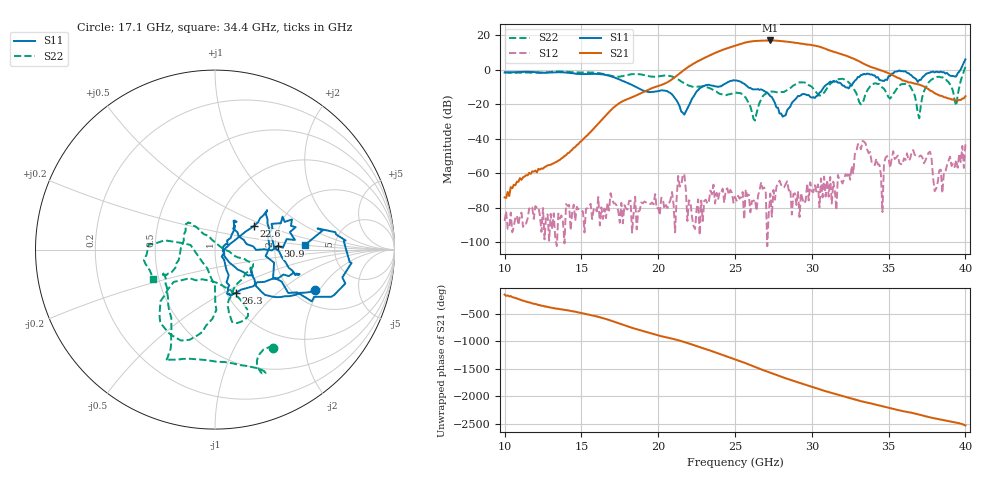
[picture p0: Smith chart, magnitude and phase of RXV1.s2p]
!Keysight Technologies,M9808A,MY58100618,A.14.70.03
!Date: Monday, February 27, 2023 13:25:10
!Correction: S11(Cdelta 2-Port  )
!S21(Cdelta 2-Port  )
!S12(Cdelta 2-Port  )
!S22(Cdelta 2-Port  )
!S2P File: Measurements: S11, S21, S12, S22:
# Hz S  RI  R 50
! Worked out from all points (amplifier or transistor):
!   301 points, 10 GHz to 40 GHz, reference 50 ohm
!   highest |S21| = 16.9 dB at 27.3 GHz (marker M1)
!   |S21| within 3 dB of that: 25.01 GHz to 30.24 GHz (5.222 GHz wide, 18.9 % of centre)
!   unconditionally stable (mu >= 1): start of sweep to 39.64 GHz
!   at 15 GHz: K = 99719.20, MAG = -32.9 dB, |S12| = -81.6 dB
!   at 25 GHz: K = 358.96, MAG = 15.2 dB, |S12| = -73.7 dB
!   at 40 GHz: K = 566.44, MSG = 14.0 dB, |S12| = -43.4 dB
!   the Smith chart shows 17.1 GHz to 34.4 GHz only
!   S11 on the Smith chart (normalised r, x): 17.1 GHz: 2.58, -1.83; 22.6 GHz: 1.48, +0.42; 26.3 GHz: 1.10, -0.57; 30.9 GHz: 2.07, +0.10; 34.4 GHz: 3.02, +0.23
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1e10  0.1017 0.8226  -0.000174 -9.79e-05  1.08e-07 -4.14e-05  0.6897 0.4632
1.5e10  0.7404 0.0739  -0.00493 -0.00703  7.26e-05 4.13e-05  0.6592 -0.495
1.71e10  0.5569 -0.2259  0.0154 0.0785  0.000134 1.4e-05  0.3258 -0.5456
2e10  0.2012 -0.1266  -0.3335 -0.0387  -8.62e-05 -5.11e-05  -0.1776 -0.6089
2.26e10  0.2175 0.1331  1.697 -0.4654  0.000171 3.16e-05  -0.293 -0.1269
2.38e10  0.3004 0.1202  -1.916 -2.506  -0.000217 0.000162  -0.2149 -0.0762
2.44e10  0.3943 -0.0725  -3.981 0.4374  -8.21e-05 0.000315  -0.1734 0.0526
2.5e10  0.4632 -0.14  -1.991 4.487  0.000167 -0.000123  -0.162 0.143
2.56e10  0.3542 -0.1585  3.627 4.68  2.11e-05 -4.07e-05  -0.1102 0.1299
2.63e10  0.1152 -0.2418  6.027 -2.932  0.000167 5.09e-05  0.029 0.0165
2.68e10  0.0669 -0.246  1.226 -6.776  0.000256 0.000241  0.1591 -0.0489
2.73e10  0.0738 -0.153  -4.599 -5.233  0.000258 8.71e-06  0.2125 -0.0834
2.79e10  0.0374 -0.0385  -6.599 1.509  -0.00022 0.000569  0.1631 -0.146
2.86e10  0.068 0.0514  -1.102 6.137  0.000209 0.000287  0.0767 -0.2795
2.93e10  0.1052 0.1503  4.523 3.402  -0.000264 4.07e-05  0.1484 -0.4008
3e10  0.1005 0.118  4.608 -2.216  7.49e-05 -0.000287  0.1446 -0.2817
3.09e10  0.3494 0.0205  -1.138 -3.815  0.000117 -0.000175  -0.1825 -0.1699
3.16e10  0.4289 0.1678  -2.961 -0.9468  7.49e-05 4.21e-05  -0.3049 -0.4081
3.25e10  0.3292 -0.0728  -1.343 1.818  -0.000563 -0.000319  -0.0147 -0.3858
3.44e10  0.5039 0.0278  0.9813 -0.094  0.00108 -0.00141  -0.3443 -0.1622
3.5e10  0.5488 -0.342  0.5272 -0.5757  0.00199 0.00188  0.0132 -0.1577
4e10  0.8796 -1.769  0.1676 -0.0248  0.00661 0.00158  0.6039 -1.041
